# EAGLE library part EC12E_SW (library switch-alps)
ALPS rotary Encoder EC12E series with switch
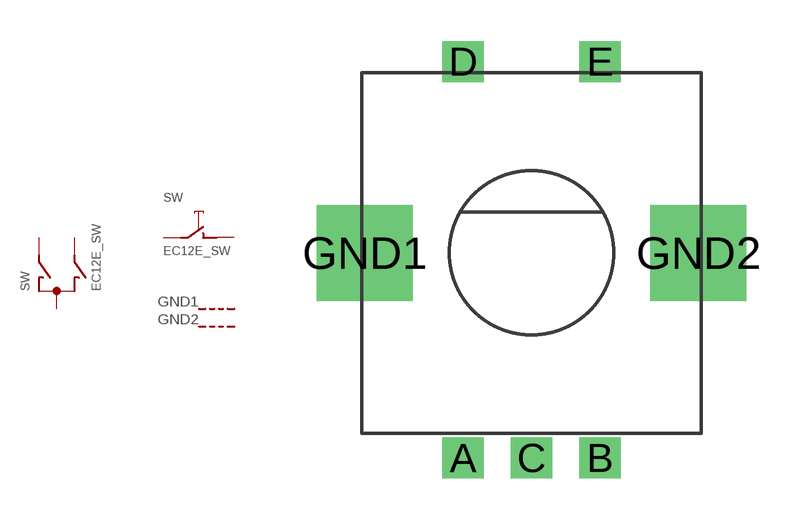
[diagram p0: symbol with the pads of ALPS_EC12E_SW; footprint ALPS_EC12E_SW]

Designator prefix SW; gates G$1=ENCODER G$2=TASTER G$3=GEHAEUSEANSCHLUSS G$4=GEHAEUSEANSCHLUSS

## EC12E_SW (MPN: EC12E2424407; OC_FARNELL: 1520813; OC_NEWARK: 74M1068)  [ALPS_EC12E_SW]
A  G$1:A  pas
B  G$1:B  pas
C  G$1:C  pas
D  G$2:1  pas
E  G$2:2  pas
GND1  G$3:G  pas
GND2  G$4:G  pas

## Footprint ALPS_EC12E_SW (pad centres in mm)
ALPS rotary encoder EC12E series with push-on switch
drill 1 square: A -2.5,-7.5; B 2.5,-7.5; C 0,-7.5; D -2.5,7; E 2.5,7
drill 2.5 square: GND1 -6.1,0; GND2 6.1,0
